| TEXAS INSTRUMENTS INCORPORATED
| Standard Linear and Logic Group
| IBIS Model of SN74ALVCH162344
| 1-BIT TO 4-BIT ADDRESS DRIVER WITH 3-STATE OUTPUTS
| This file contains package information for the following:
|  SSOP 56-pin (DL) package as [Component] ALVCH162344_DL
|  TSSOP 56-pin (DGG) package as [Component] ALVCH162344_DGG
|  TVSOP 56-pin (DGV) package as [Component] ALVCH162344_DGV
| This device can be powered at the following Vccs:
|  3.3 volt Vcc
|  2.5 volt Vcc
|  1.8 volt Vcc
| This file provides unique models under the [Model Selector] for each Vcc.
| For operation at a specific Vcc, select the appropriate model after each
| [Model Selector] keyword.
[IBIS Ver]   3.2
[Comment char]  |_char
[File Name]   sn74alvch162344.ibs
[File Rev]   1.1 | x_die
[Date]   Sept 13, 2001
[Source]   Data created from TI-SPICE simulations at TI-SLL.
[Notes]   The following is an IBIS list for the ALVCH162344.
   Please contact sllibis@ti.com with questions and
   comments concerning SLL IBIS models.
   Non-Convergence in the following files:
   gc_alvch162344_oein_33, extrapolated from 0.5 V plus
   pc_alvch162344_oein_33, extrapolated from 0.93 V plus
   gc_alvch162344_oein_25, extrapolated from 0.5 V plus
   pc_alvch162344_oein_25, extrapolated from 0.69 V plus
   gc_alvch162344_oein_18, extrapolated from 0.5 V plus
   pc_alvch162344_oein_18, extrapolated from 0.5 V plus
   - Due to Bus Hold in the input circuit, some Clamp curves
   have non-monotonic data
[Disclaimer] Property of Texas Instruments Incorporated.  Unauthorized
   reproduction and/or distribution is strictly prohibited.
   This product is protected under copyright law.
   Created  2001, (C) Copyright  2001, Texas Instruments
   Incorporated, All Rights Reserved
   UNLESS THERE IS A SIGNED, WRITTEN AGREEMENT TO THE
   CONTRARY, TEXAS INSTRUMENTS (TI) IS PROVIDING THE IBIS
   MODELS  AND WITHOUT ANY WARRANTY, EXPRESSED OR
   IMPLIED.  TI assumes no liability for:
   1) the accuracy of the IBIS models provided to your
   company;
   2) the proper functioning of these IBIS Models in your
   design or for any resulting applications; or
   3) infringement of patents, copyrights or intellectual
   property rights resulting from your use of these IBIS
   models.
   TI provides IBIS Models as a service to our customers.
   You and your company shall not distribute, sell or give
   these models to anyone else without prior written
   permission from TI.
   TI reserves the right to make changes to our products or
   to discontinue any semiconductor product or service
   without notice, and advises our customers to obtain the
   latest version of relevant information to verify, before
   placing orders, that the information being relied on is
   current.
   Please be aware that your receipt and use of the IBIS
   information provided shall serve as acceptance of these
   terms and conditions.  If you do not accept these terms,
   you should return or destroy the IBIS models and any
   other accompanying information immediately.
| Component ALVCH162344_DL 56-pin SSOP
[Component]   ALVCH162344_DL
[Manufacturer]   Texas Instruments, Inc.
[Package]
|   typ   min   max
R_pkg   5.500e-02   4.800e-02   6.700e-02
L_pkg   6.539e-09   4.802e-09   9.746e-09
C_pkg   1.880e-13   7.600e-14   5.170e-13
[Pin]   signal_name   model_name   R_pin   L_pin   C_pin
1   NOE1   ALVCH162344_OEIN   6.400e-02   9.646e-09   5.130e-13
2   1B1   ALVCH162344_OUT   5.900e-02   8.723e-09   2.700e-13
3   1B2   ALVCH162344_OUT   5.900e-02   8.139e-09   2.230e-13
4   GND   GND   5.600e-02   7.554e-09   2.010e-13
5   1B3   ALVCH162344_OUT   5.400e-02   6.991e-09   1.950e-13
6   1B4   ALVCH162344_OUT   5.300e-02   6.659e-09   2.020e-13
7   VCC   POWER   5.500e-02   6.321e-09   2.070e-13
8   1A   ALVCH162344_IN   5.500e-02   5.942e-09   1.330e-13
9   2B1   ALVCH162344_OUT   5.700e-02   5.767e-09   1.320e-13
10   2B2   ALVCH162344_OUT   5.400e-02   5.459e-09   1.210e-13
11   GND   GND   5.100e-02   5.224e-09   1.400e-13
12   2B3   ALVCH162344_OUT   4.800e-02   5.088e-09   1.260e-13
13   2B4   ALVCH162344_OUT   5.000e-02   5.021e-09   9.600e-14
14   2A   ALVCH162344_IN   5.100e-02   4.802e-09   7.600e-14
15   3A   ALVCH162344_IN   5.100e-02   4.803e-09   7.600e-14
16   3B1   ALVCH162344_OUT   5.000e-02   5.021e-09   9.600e-14
17   3B2   ALVCH162344_OUT   4.800e-02   5.088e-09   1.260e-13
18   GND   GND   5.100e-02   5.224e-09   1.400e-13
19   3B3   ALVCH162344_OUT   5.400e-02   5.459e-09   1.210e-13
20   3B4   ALVCH162344_OUT   5.700e-02   5.768e-09   1.330e-13
21   4A   ALVCH162344_IN   5.500e-02   5.942e-09   1.330e-13
22   VCC   POWER   5.500e-02   6.320e-09   2.060e-13
23   4B1   ALVCH162344_OUT   5.300e-02   6.659e-09   2.030e-13
24   4B2   ALVCH162344_OUT   5.400e-02   6.991e-09   1.960e-13
25   GND   GND   5.600e-02   7.554e-09   2.010e-13
26   4B3   ALVCH162344_OUT   5.900e-02   8.139e-09   2.230e-13
27   4B4   ALVCH162344_OUT   5.900e-02   8.727e-09   2.700e-13
28   NOE2   ALVCH162344_OEIN   6.700e-02   9.746e-09   5.170e-13
29   NOE3   ALVCH162344_OEIN   6.300e-02   9.630e-09   5.110e-13
30   5B4   ALVCH162344_OUT   6.000e-02   8.751e-09   2.710e-13
31   5B3   ALVCH162344_OUT   6.000e-02   8.184e-09   2.250e-13
32   GND   GND   5.600e-02   7.543e-09   2.000e-13
33   5B2   ALVCH162344_OUT   5.400e-02   7.005e-09   1.960e-13
34   5B1   ALVCH162344_OUT   5.600e-02   6.714e-09   2.040e-13
35   VCC   POWER   5.800e-02   6.384e-09   2.080e-13
36   5A   ALVCH162344_IN   5.700e-02   5.976e-09   1.340e-13
37   6B4   ALVCH162344_OUT   5.700e-02   5.743e-09   1.300e-13
38   6B3   ALVCH162344_OUT   5.400e-02   5.468e-09   1.190e-13
39   GND   GND   5.500e-02   5.328e-09   1.420e-13
40   6B2   ALVCH162344_OUT   5.200e-02   5.189e-09   1.290e-13
41   6B1   ALVCH162344_OUT   5.200e-02   5.053e-09   9.600e-14
42   6A   ALVCH162344_IN   5.100e-02   4.825e-09   7.600e-14
43   7A   ALVCH162344_IN   5.400e-02   4.896e-09   7.800e-14
44   7B4   ALVCH162344_OUT   5.200e-02   5.093e-09   9.700e-14
45   7B3   ALVCH162344_OUT   5.100e-02   5.179e-09   1.280e-13
46   GND   GND   5.400e-02   5.314e-09   1.420e-13
47   7B2   ALVCH162344_OUT   5.500e-02   5.511e-09   1.210e-13
48   7B1   ALVCH162344_OUT   5.700e-02   5.771e-09   1.310e-13
49   8A   ALVCH162344_IN   5.600e-02   5.957e-09   1.330e-13
50   VCC   POWER   5.500e-02   6.320e-09   2.060e-13
51   8B4   ALVCH162344_OUT   5.200e-02   6.621e-09   2.000e-13
52   8B3   ALVCH162344_OUT   5.300e-02   6.973e-09   1.950e-13
53   GND   GND   5.700e-02   7.571e-09   2.020e-13
54   8B2   ALVCH162344_OUT   5.700e-02   8.097e-09   2.220e-13
55   8B1   ALVCH162344_OUT   5.900e-02   8.723e-09   2.710e-13
56   NOE4   ALVCH162344_OEIN   6.100e-02   9.560e-09   5.090e-13
| Component ALVCH162344_DGG 56-pin TSSOP
[Component]   ALVCH162344_DGG
[Manufacturer]   Texas Instruments, Inc.
[Package]
|   typ   min   max
R_pkg   4.500e-02   3.500e-02   6.200e-02
L_pkg   3.324e-09   2.403e-09   5.094e-09
C_pkg   5.640e-13   3.410e-13   9.140e-13
[Pin]   signal_name   model_name   R_pin   L_pin   C_pin
1   NOE1   ALVCH162344_OEIN   6.200e-02   5.094e-09   8.560e-13
2   1B1   ALVCH162344_OUT   6.100e-02   4.621e-09   9.020e-13
3   1B2   ALVCH162344_OUT   6.000e-02   4.316e-09   8.020e-13
4   GND   GND   5.900e-02   3.968e-09   6.980e-13
5   1B3   ALVCH162344_OUT   5.700e-02   3.716e-09   6.490e-13
6   1B4   ALVCH162344_OUT   4.200e-02   3.517e-09   6.520e-13
7   VCC   POWER   4.100e-02   3.160e-09   5.700e-13
8   1A   ALVCH162344_IN   3.900e-02   2.981e-09   4.820e-13
9   2B1   ALVCH162344_OUT   3.900e-02   2.809e-09   4.470e-13
10   2B2   ALVCH162344_OUT   3.800e-02   2.715e-09   4.090e-13
11   GND   GND   4.100e-02   2.675e-09   3.910e-13
12   2B3   ALVCH162344_OUT   3.900e-02   2.536e-09   3.660e-13
13   2B4   ALVCH162344_OUT   3.900e-02   2.457e-09   3.480e-13
14   2A   ALVCH162344_IN   3.800e-02   2.411e-09   3.530e-13
15   3A   ALVCH162344_IN   3.900e-02   2.456e-09   3.550e-13
16   3B1   ALVCH162344_OUT   3.900e-02   2.471e-09   3.490e-13
17   3B2   ALVCH162344_OUT   4.000e-02   2.580e-09   3.700e-13
18   GND   GND   3.800e-02   2.651e-09   3.890e-13
19   3B3   ALVCH162344_OUT   3.800e-02   2.739e-09   4.110e-13
20   3B4   ALVCH162344_OUT   3.900e-02   2.838e-09   4.490e-13
21   4A   ALVCH162344_IN   3.800e-02   2.988e-09   4.840e-13
22   VCC   POWER   3.800e-02   3.105e-09   5.640e-13
23   4B1   ALVCH162344_OUT   4.000e-02   3.427e-09   6.380e-13
24   4B2   ALVCH162344_OUT   5.600e-02   3.654e-09   6.410e-13
25   GND   GND   5.700e-02   3.932e-09   7.000e-13
26   4B3   ALVCH162344_OUT   5.800e-02   4.257e-09   8.060e-13
27   4B4   ALVCH162344_OUT   5.700e-02   4.580e-09   9.140e-13
28   NOE2   ALVCH162344_OEIN   5.900e-02   5.038e-09   8.610e-13
29   NOE3   ALVCH162344_OEIN   6.000e-02   5.058e-09   8.580e-13
30   5B4   ALVCH162344_OUT   5.600e-02   4.543e-09   9.040e-13
31   5B3   ALVCH162344_OUT   5.700e-02   4.240e-09   8.030e-13
32   GND   GND   5.700e-02   3.929e-09   7.000e-13
33   5B2   ALVCH162344_OUT   5.600e-02   3.616e-09   6.370e-13
34   5B1   ALVCH162344_OUT   3.700e-02   3.368e-09   6.400e-13
35   VCC   POWER   3.600e-02   3.024e-09   5.630e-13
36   5A   ALVCH162344_IN   3.500e-02   2.876e-09   4.740e-13
37   6B4   ALVCH162344_OUT   3.500e-02   2.745e-09   4.440e-13
38   6B3   ALVCH162344_OUT   3.700e-02   2.683e-09   4.050e-13
39   GND   GND   3.800e-02   2.603e-09   3.820e-13
40   6B2   ALVCH162344_OUT   3.800e-02   2.510e-09   3.620e-13
41   6B1   ALVCH162344_OUT   3.600e-02   2.412e-09   3.410e-13
42   6A   ALVCH162344_IN   3.800e-02   2.416e-09   3.490e-13
43   7A   ALVCH162344_IN   3.700e-02   2.403e-09   3.490e-13
44   7B4   ALVCH162344_OUT   3.700e-02   2.429e-09   3.410e-13
45   7B3   ALVCH162344_OUT   3.600e-02   2.482e-09   3.580e-13
46   GND   GND   3.700e-02   2.615e-09   3.810e-13
47   7B2   ALVCH162344_OUT   3.500e-02   2.669e-09   4.020e-13
48   7B1   ALVCH162344_OUT   3.600e-02   2.763e-09   4.420e-13
49   8A   ALVCH162344_IN   3.600e-02   2.942e-09   4.780e-13
50   VCC   POWER   3.500e-02   3.053e-09   5.640e-13
51   8B4   ALVCH162344_OUT   3.600e-02   3.409e-09   6.410e-13
52   8B3   ALVCH162344_OUT   5.800e-02   3.698e-09   6.410e-13
53   GND   GND   5.900e-02   3.975e-09   6.970e-13
54   8B2   ALVCH162344_OUT   6.100e-02   4.327e-09   8.020e-13
55   8B1   ALVCH162344_OUT   6.100e-02   4.624e-09   9.050e-13
56   NOE4   ALVCH162344_OEIN   6.000e-02   5.063e-09   8.580e-13
| Component ALVCH162344_DGV 56-pin TVSOP
[Component]   ALVCH162344_DGV
[Manufacturer]   Texas Instruments, Inc.
[Package]
|   typ   min   max
R_pkg   6.300e-02   5.000e-02   8.600e-02
L_pkg   2.945e-09   2.392e-09   3.938e-09
C_pkg   3.910e-13   2.710e-13   5.880e-13
[Pin]   signal_name   model_name   R_pin   L_pin   C_pin
1   NOE1   ALVCH162344_OEIN   6.800e-02   3.933e-09   5.880e-13
2   1B1   ALVCH162344_OUT   6.800e-02   3.569e-09   5.860e-13
3   1B2   ALVCH162344_OUT   7.600e-02   3.464e-09   5.150e-13
4   GND   GND   8.600e-02   3.451e-09   4.580e-13
5   1B3   ALVCH162344_OUT   8.200e-02   3.278e-09   4.260e-13
6   1B4   ALVCH162344_OUT   7.700e-02   3.143e-09   3.870e-13
7   VCC   POWER   6.900e-02   2.971e-09   4.010e-13
8   1A   ALVCH162344_IN   5.000e-02   2.787e-09   3.790e-13
9   2B1   ALVCH162344_OUT   5.100e-02   2.686e-09   3.200e-13
10   2B2   ALVCH162344_OUT   5.200e-02   2.607e-09   3.160e-13
11   GND   GND   5.300e-02   2.497e-09   2.970e-13
12   2B3   ALVCH162344_OUT   5.400e-02   2.438e-09   2.920e-13
13   2B4   ALVCH162344_OUT   5.500e-02   2.412e-09   2.860e-13
14   2A   ALVCH162344_IN   5.500e-02   2.400e-09   2.730e-13
15   3A   ALVCH162344_IN   5.500e-02   2.402e-09   2.730e-13
16   3B1   ALVCH162344_OUT   5.400e-02   2.398e-09   2.840e-13
17   3B2   ALVCH162344_OUT   5.400e-02   2.407e-09   2.890e-13
18   GND   GND   5.300e-02   2.448e-09   2.930e-13
19   3B3   ALVCH162344_OUT   5.200e-02   2.548e-09   3.110e-13
20   3B4   ALVCH162344_OUT   5.100e-02   2.623e-09   3.160e-13
21   4A   ALVCH162344_IN   5.000e-02   2.725e-09   3.700e-13
22   VCC   POWER   6.500e-02   2.903e-09   3.940e-13
23   4B1   ALVCH162344_OUT   7.300e-02   3.086e-09   3.870e-13
24   4B2   ALVCH162344_OUT   8.200e-02   3.272e-09   4.280e-13
25   GND   GND   8.200e-02   3.394e-09   4.570e-13
26   4B3   ALVCH162344_OUT   7.100e-02   3.374e-09   5.080e-13
27   4B4   ALVCH162344_OUT   6.900e-02   3.572e-09   5.810e-13
28   NOE2   ALVCH162344_OEIN   6.900e-02   3.937e-09   5.740e-13
29   NOE3   ALVCH162344_OEIN   6.900e-02   3.923e-09   5.690e-13
30   5B4   ALVCH162344_OUT   6.800e-02   3.546e-09   5.740e-13
31   5B3   ALVCH162344_OUT   7.400e-02   3.422e-09   5.180e-13
32   GND   GND   8.100e-02   3.395e-09   4.680e-13
33   5B2   ALVCH162344_OUT   8.000e-02   3.255e-09   4.310e-13
34   5B1   ALVCH162344_OUT   7.100e-02   3.063e-09   3.860e-13
35   VCC   POWER   6.100e-02   2.878e-09   3.900e-13
36   5A   ALVCH162344_IN   5.000e-02   2.709e-09   3.640e-13
37   6B4   ALVCH162344_OUT   5.100e-02   2.607e-09   3.110e-13
38   6B3   ALVCH162344_OUT   5.100e-02   2.532e-09   3.060e-13
39   GND   GND   5.300e-02   2.440e-09   2.890e-13
40   6B2   ALVCH162344_OUT   5.300e-02   2.399e-09   2.860e-13
41   6B1   ALVCH162344_OUT   5.400e-02   2.392e-09   2.820e-13
42   6A   ALVCH162344_IN   5.500e-02   2.399e-09   2.710e-13
43   7A   ALVCH162344_IN   5.500e-02   2.395e-09   2.710e-13
44   7B4   ALVCH162344_OUT   5.500e-02   2.403e-09   2.830e-13
45   7B3   ALVCH162344_OUT   5.400e-02   2.421e-09   2.880e-13
46   GND   GND   5.300e-02   2.472e-09   2.920e-13
47   7B2   ALVCH162344_OUT   5.100e-02   2.569e-09   3.090e-13
48   7B1   ALVCH162344_OUT   5.100e-02   2.636e-09   3.130e-13
49   8A   ALVCH162344_IN   5.000e-02   2.739e-09   3.660e-13
50   VCC   POWER   6.500e-02   2.922e-09   3.900e-13
51   8B4   ALVCH162344_OUT   7.200e-02   3.076e-09   3.840e-13
52   8B3   ALVCH162344_OUT   8.100e-02   3.249e-09   4.300e-13
53   GND   GND   8.300e-02   3.400e-09   4.550e-13
54   8B2   ALVCH162344_OUT   7.300e-02   3.421e-09   5.060e-13
55   8B1   ALVCH162344_OUT   6.900e-02   3.579e-09   5.780e-13
56   NOE4   ALVCH162344_OEIN   6.900e-02   3.938e-09   5.810e-13
| Model ALVCH162344_IN
[Model Selector]   ALVCH162344_IN
ALVCH162344_IN_33   3.3 volt Vcc
ALVCH162344_IN_25   2.5 volt Vcc
ALVCH162344_IN_18   1.8 volt Vcc
| Model ALVCH162344_OEIN
[Model Selector]   ALVCH162344_OEIN
ALVCH162344_OEIN_33   3.3 volt Vcc
ALVCH162344_OEIN_25   2.5 volt Vcc
ALVCH162344_OEIN_18   1.8 volt Vcc
| Model ALVCH162344_OUT
[Model Selector]   ALVCH162344_OUT
ALVCH162344_OUT_33   3.3 volt Vcc
ALVCH162344_OUT_25   2.5 volt Vcc
ALVCH162344_OUT_18   1.8 volt Vcc
| Models and submodels in the file (9): ALVCH162344_IN_33 (Input), ALVCH162344_IN_25 (Input), ALVCH162344_IN_18 (Input), ALVCH162344_OEIN_33 (Input), ALVCH162344_OEIN_25 (Input), ALVCH162344_OEIN_18 (Input), ALVCH162344_OUT_33 (3-state), ALVCH162344_OUT_25 (3-state), ALVCH162344_OUT_18 (3-state)
